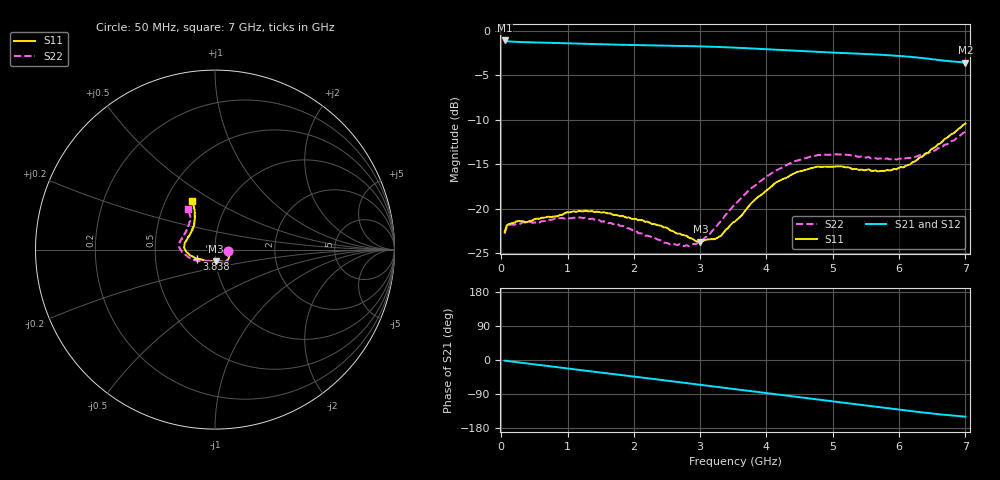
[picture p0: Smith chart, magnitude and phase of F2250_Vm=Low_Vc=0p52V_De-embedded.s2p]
! Integrated Device Technology
! Corporate Headquarters
! 6024 Silver Creek Valley Road
! San Jose, CA 95138  USA
! Phone:  1-408-284-8200
! Toll Free:  1-800-223-1366
! Webpage:  http://www.idt.com/
! Timing and RF Division
! 515 Groton Road, Suite 102
! Westford, MA 01886-6024
! Device:  F2250
! Description: Voltage Variable RF Attenuator
! Frequency:  50.0 -  6000.00 MHz
! Package:  3x3 mm Thin QFN Plastic Package: 16 pin
! Ports:  2 RF, 3 DC
!  Pin  1  = GND
!  Pin  2  = NC
!  Pin  3  = RF1  = Port 1
!  Pin  4  = NC
!  Pin  5  = GND
!  Pin  6  = GND
!  Pin  7  = GND
!  Pin  8  = GND
!  Pin  9  = NC
!  Pin 10  = RF2  = Port 2
!  Pin 11  = NC
!  Pin 12  = GND
!  Pin 13  = GND
!  Pin 14  = VCNTRL
!  Pin 15  = VDD
!  Pin 16  = VMODE
! Vcntrl:  0.520 Volts
! Vmode:  +0.000 Volts
! Vdd:  +3.30  Volts
! Current:  1.132 mA
! Data:  The device was measured on a the F2250 evaluation board which has
!  individual transmission lines to the RF pins.  Data was collected
!  using a calibrated network analyzer.  The evaluation board was
!  de-embedded using a TRL calibration technique.
!  The reference plane is the edge of the package pin.
! Misc:  SN 10
!  Action Tracker AT0258
! Date Measured:  2014-11-26
! Date:  2015-10-15  MJV
! Note:
!  Integrated Device Technology supplies this data as a sample of measured
!  data at the package pin for this product.  Your particular data for this
!  product may vary.
!  Data was taken at 25 degrees C.
!  Integrated Device Technology reserves the right to change this data at anytime.
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# GHz S dB R 50
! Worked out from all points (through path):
!   201 points, 50 MHz to 7 GHz, reference 50 ohm
!   highest |S21| = -1.11 dB at 50 MHz (marker M1); lowest = -3.6 dB at 7 GHz (marker M2)
!   group delay of S21, straight-line fit = 60.1 ps
!   lowest |S11| = -23.7 dB at 3.004 GHz (marker M3), VSWR 1.14, Z = 49.9 - j6.54 ohm
!   |S11| at or under -10 dB: start of sweep to end of sweep
!   |S22| runs from -24.2 to -11.3 dB; largest |S21 - S12| = 0.00041
!   S11 on the Smith chart (normalised r, x): 50 MHz: 1.16, -0.02; 3.838 GHz: 0.81, -0.08; 7 GHz: 0.68, +0.40
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0.05  -22.63 -7.4  -1.11 -1.8  -1.10 -1.8  -22.82 -8.4
0.08475  -21.86 -7.5  -1.19 -2.5  -1.19 -2.5  -22.00 -7.8
0.15425  -21.64 -9.6  -1.24 -4.0  -1.24 -4.0  -21.77 -9.6
0.6755  -20.96 -30.5  -1.37 -15.4  -1.36 -15.4  -21.38 -33.0
1.2315  -20.31 -48.7  -1.49 -27.4  -1.48 -27.4  -21.07 -55.3
1.75275  -20.74 -55.4  -1.58 -38.5  -1.58 -38.5  -21.72 -64.1
2.37825  -21.88 -57.4  -1.67 -51.8  -1.67 -51.8  -23.51 -70.5
2.7605  -23.00 -69.2  -1.73 -60.2  -1.73 -60.2  -24.21 -87.5
3.00375  -23.70 -87.1  -1.77 -65.6  -1.77 -65.6  -23.58 -106.7
3.14275  -23.44 -98.6  -1.80 -68.6  -1.80 -68.6  -22.87 -118.4
3.3165  -23.03 -117.6  -1.85 -72.5  -1.85 -72.5  -21.38 -130.3
3.525  -21.44 -135.1  -1.91 -77.2  -1.91 -77.2  -19.55 -142.4
3.83775  -18.92 -153.8  -2.03 -84.1  -2.03 -84.1  -17.36 -156.6
4.1505  -17.02 -166.5  -2.15 -90.9  -2.16 -90.9  -15.68 -168.8
4.4285  -15.99 -174.9  -2.26 -97.0  -2.26 -97.0  -14.66 -176.3
4.7065  -15.40 178.0  -2.37 -103.0  -2.37 -103.0  -14.12 177.4
5.15825  -15.29 167.0  -2.53 -112.7  -2.53 -112.7  -13.88 167.9
5.85325  -15.71 143.4  -2.77 -127.6  -2.77 -127.7  -14.46 152.3
6.166  -15.04 131.7  -2.94 -134.4  -2.94 -134.5  -14.31 143.3
6.444  -13.69 122.6  -3.15 -140.2  -3.15 -140.3  -13.76 133.8
6.82625  -11.52 116.2  -3.47 -146.9  -3.47 -146.9  -12.34 125.7
7  -10.44 115.3  -3.59 -149.6  -3.59 -149.6  -11.34 124.2
